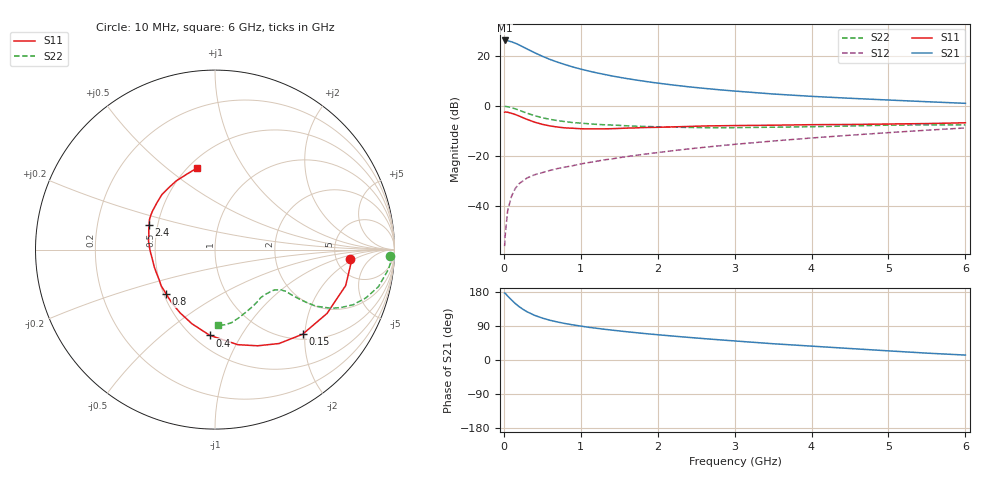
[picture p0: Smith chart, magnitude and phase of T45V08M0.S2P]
! Infineon Technologies  Discrete & RF Semiconductors
! BFR182T
! Si NPN RF Bipolar Junction Transistor in SC75
! VCE = 5 V  IC = 8 mA
! Common Emitter S-Parameters:  October  1999
# GHz  S  MA  R  50
!  f  S11  S21  S12  S22
! GHz  MAG  ANG  MAG  ANG  MAG  ANG  MAG  ANG
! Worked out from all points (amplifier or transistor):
!   36 points, 10 MHz to 6 GHz, reference 50 ohm
!   highest |S21| = 26.2 dB at 10 MHz (marker M1)
!   |S21| within 3 dB of that: start of sweep to 275.7 MHz
!   unconditionally stable (mu >= 1): 1.162 GHz to 3.91 GHz
!   at 250 MHz: K = 0.38, MSG = 26.7 dB, |S12| = -29.8 dB
!   at 1.4 GHz: K = 1.05, MAG = 15.2 dB, |S12| = -21.1 dB
!   at 6 GHz: K = 0.85, MSG = 4.9 dB, |S12| = -8.7 dB
!   lowest NFmin = 1.40 dB at 450 MHz
!   S11 on the Smith chart (normalised r, x): 10 MHz: 6.71, -1.68; 150 MHz: 1.11, -1.95; 400 MHz: 0.60, -0.74; 800 MHz: 0.51, -0.29; 2.4 GHz: 0.45, +0.15; 6 GHz: 0.55, +0.64
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0.01  0.7544 -4.1  20.47 176.7  0.0016 85.3  0.9768 -2.0
0.02  0.7632 -4.8  20.42 175.5  0.0029 83.5  0.989 -2.7
0.05  0.7552 -15.4  20.21 168.7  0.0082 84.3  0.9711 -6.7
0.1  0.7183 -29.7  19.25 158.5  0.0159 76.2  0.9337 -12.8
0.15  0.6786 -44.0  18.02 148.7  0.0229 69.9  0.882 -17.8
0.2  0.6335 -55.7  16.64 140.6  0.0284 66.6  0.8281 -21.8
0.25  0.5861 -66.1  15.18 133.6  0.0323 62.7  0.7725 -24.7
0.3  0.5448 -76.5  13.87 127.5  0.0367 60.3  0.725 -26.8
0.4  0.4789 -93.4  11.65 117.8  0.0427 57.4  0.6439 -29.3
0.5  0.433 -107.2  9.912 110.7  0.047 57.0  0.587 -30.0
0.6  0.4023 -119.0  8.558 104.8  0.0521 56.7  0.5447 -30.4
0.7  0.3817 -129.3  7.535 100.2  0.0568 57.7  0.5129 -30.5
0.8  0.3673 -137.9  6.72 96.1  0.0608 58.1  0.4892 -30.6
1.1  0.3511 -158.8  5.032 86.4  0.0745 60.3  0.445 -31.0
1.3  0.3522 -169.0  4.318 81.3  0.0844 61.7  0.4251 -31.9
1.6  0.3644 178.8  3.549 74.5  0.0983 62.9  0.4047 -33.6
2.2  0.3854 163.3  2.639 63.1  0.129 64.4  0.3812 -39.5
2.4  0.3924 159.2  2.435 59.7  0.1397 64.5  0.3747 -41.8
3.5  0.4161 140.8  1.747 42.9  0.2011 62.7  0.3795 -55.8
4.5  0.4301 127.3  1.435 30.3  0.2626 58.9  0.4012 -70.2
5.5  0.4486 110.5  1.225 18.1  0.3309 53.8  0.4223 -82.6
6  0.4651 102.4  1.137 13.0  0.3668 50.3  0.4223 -87.8
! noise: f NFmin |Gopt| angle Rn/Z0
0.45  1.4  0.26  41  0.29
0.9  1.5  0.25  83  0.23
1.8  2  0.21  162  0.2
